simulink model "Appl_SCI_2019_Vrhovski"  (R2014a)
settings: Solver=ode45  StartTime=0.0  StopTime=1000  MaxStep=0.01  RelTol=1e-3
undefined symbols (not defined in the file): deg, H, kg, m, M, mm, N, rad, s, X, Y, Z
libraries: sm_lib x389, nesl_utility x69, simulink x7
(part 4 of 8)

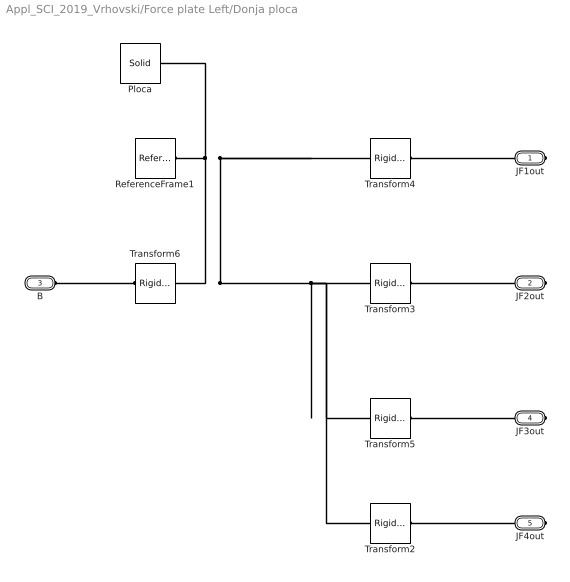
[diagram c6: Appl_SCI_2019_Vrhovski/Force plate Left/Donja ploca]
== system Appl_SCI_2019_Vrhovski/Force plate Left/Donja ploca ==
  Ploca : sm_lib/Body Elements/Solid  InertiaType=Custom  Mass=3.25  MassUnits=kg  CenterOfMass=[0 0 0]  CenterOfMassUnits=mm  MomentsOfInertia=[7450 490 7450]  MomentsOfInertiaUnits=kg*mm^2  ProductsOfInertia=[0 0 0]  ProductsOfInertiaUnits=kg*mm^2  DensityBased=on  Density=1000  DensityUnits=kg/(m^3)  GraphicType=FromGeometry  MarkerShape=Sphere  MarkerSize=10  MarkerSizeUnits=m  GraphicVisPropType=SimpleVisualProperties  GraphicDiffuseColor=[0.6 0.6 0.6]  GraphicSpecularColor=[0.5 0.5 0.5 1.0]  GraphicAmbientColor=[0.15 0.15 0.15 1.0]  GraphicEmissiveColor=[0.0 0.0 0.0 1.0]  GraphicShininess=75  GraphicOpacity=1  GeometryShape=Brick  RectangleSize=[1 1]  RectangleSizeUnits=m  BrickDimensions="[210  380 1]"  BrickDimensionUnits=mm  CylinderRadius=1  CylinderRadiusUnits=m  CylinderLength=1  CylinderLengthUnits=m  SphereRadius=1  SphereRadiusUnits=m  EllipsoidRadii=[1 1 1]  EllipsoidRadiiUnits=m  ExtrusionCrossSection=[1 1; -1 1; -1 -1; 1 -1]  ExtrusionCrossSectionUnits=m  ExtrusionLength=1  ExtrusionLengthUnits=m  PolygonNumSides=3  PolygonOuterRadius=1  PolygonOuterRadiusUnits=m  ExtGeomFileType=STL  ExtGeomFileName=Tijelo_Default_sldprt.STL  ExtGeomFileUnits=mm  RevolutionCrossSection=[1 1; 1 -1; 2 -1; 2 1]  RevolutionCrossSectionUnits=m  RevolutionExtent=Full  RevolutionAngle=180  RevolutionAngleUnits=deg  BlockFunction=simmechanics.library.body_elements.solid
  ReferenceFrame1 : sm_lib/Frames and Transforms/Reference Frame  BlockFunction=simmechanics.library.frames_transforms.reference_frame
  Transform2 : sm_lib/Frames and Transforms/Rigid Transform  TranslationMethod=Cartesian  TranslationLengthUnit=mm  TranslationStandardAxis=+Z  TranslationStandardOffset=15  TranslationCartesianOffset=[84 180.5 1]  TranslationROffset=0  TranslationROffsetUnits=m  TranslationZOffset=0  TranslationZOffsetUnits=m  TranslationThetaOffset=0  TranslationThetaOffsetUnits=deg  RotationMethod=None  RotationAngleUnits=rad  RotationStandardAxis=+Z  RotationAngle=2.0943951023931953  RotationArbitraryAxis=[-0.57735026918962584 -0.57735026918962584 -0.57735026918962584]  FollAlignAxisA=+X  BaseAlignAxisA=+Y  FollAlignAxisB=+Y  BaseAlignAxisB=+Z  BlockFunction=simmechanics.library.frames_transforms.rigid_transform
  Transform3 : sm_lib/Frames and Transforms/Rigid Transform  TranslationMethod=Cartesian  TranslationLengthUnit=mm  TranslationStandardAxis=+Z  TranslationStandardOffset=15  TranslationCartesianOffset=[84 -180.5 1]  TranslationROffset=0  TranslationROffsetUnits=m  TranslationZOffset=0  TranslationZOffsetUnits=m  TranslationThetaOffset=0  TranslationThetaOffsetUnits=deg  RotationMethod=None  RotationAngleUnits=rad  RotationStandardAxis=+Z  RotationAngle=2.0943951023931953  RotationArbitraryAxis=[-0.57735026918962584 -0.57735026918962584 -0.57735026918962584]  FollAlignAxisA=+X  BaseAlignAxisA=+Y  FollAlignAxisB=+Y  BaseAlignAxisB=+Z  BlockFunction=simmechanics.library.frames_transforms.rigid_transform
  Transform4 : sm_lib/Frames and Transforms/Rigid Transform  TranslationMethod=Cartesian  TranslationLengthUnit=mm  TranslationStandardAxis=+Z  TranslationStandardOffset=15  TranslationCartesianOffset=[-84 -180.5 1]  TranslationROffset=0  TranslationROffsetUnits=m  TranslationZOffset=0  TranslationZOffsetUnits=m  TranslationThetaOffset=0  TranslationThetaOffsetUnits=deg  RotationMethod=None  RotationAngleUnits=rad  RotationStandardAxis=+Z  RotationAngle=2.0943951023931953  RotationArbitraryAxis=[-0.57735026918962584 -0.57735026918962584 -0.57735026918962584]  FollAlignAxisA=+X  BaseAlignAxisA=+Y  FollAlignAxisB=+Y  BaseAlignAxisB=+Z  BlockFunction=simmechanics.library.frames_transforms.rigid_transform
  Transform5 : sm_lib/Frames and Transforms/Rigid Transform  TranslationMethod=Cartesian  TranslationLengthUnit=mm  TranslationStandardAxis=+Z  TranslationStandardOffset=15  TranslationCartesianOffset=[-84 180.5 1]  TranslationROffset=0  TranslationROffsetUnits=m  TranslationZOffset=0  TranslationZOffsetUnits=m  TranslationThetaOffset=0  TranslationThetaOffsetUnits=deg  RotationMethod=None  RotationAngleUnits=rad  RotationStandardAxis=+Z  RotationAngle=2.0943951023931953  RotationArbitraryAxis=[-0.57735026918962584 -0.57735026918962584 -0.57735026918962584]  FollAlignAxisA=+X  BaseAlignAxisA=+Y  FollAlignAxisB=+Y  BaseAlignAxisB=+Z  BlockFunction=simmechanics.library.frames_transforms.rigid_transform
  Transform6 : sm_lib/Frames and Transforms/Rigid Transform  TranslationMethod=None  TranslationLengthUnit=mm  TranslationStandardAxis=+Z  TranslationStandardOffset=15  TranslationCartesianOffset="[50  50 15]"  TranslationROffset=0  TranslationROffsetUnits=m  TranslationZOffset=0  TranslationZOffsetUnits=m  TranslationThetaOffset=0  TranslationThetaOffsetUnits=deg  RotationMethod=None  RotationAngleUnits=rad  RotationStandardAxis=+Z  RotationAngle=2.0943951023931953  RotationArbitraryAxis=[-0.57735026918962584 -0.57735026918962584 -0.57735026918962584]  FollAlignAxisA=+X  BaseAlignAxisA=+Y  FollAlignAxisB=+Y  BaseAlignAxisB=+Z  BlockFunction=simmechanics.library.frames_transforms.rigid_transform
  JF1out : PMIOPort  Port=1  Side=Right
  JF2out : PMIOPort  Port=2  Side=Right
  B : PMIOPort  Port=3  Side=Left
  JF3out : PMIOPort  Port=4  Side=Right
  JF4out : PMIOPort  Port=5  Side=Right
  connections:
  JF1out/RConn1 -- Transform4/RConn1
  JF4out/RConn1 -- Transform2/RConn1
  JF3out/RConn1 -- Transform5/RConn1
  ReferenceFrame1/RConn1 -- Ploca/RConn1 -- Transform4/LConn1 -- Transform2/LConn1 -- Transform5/LConn1 -- Transform3/LConn1 -- Transform6/LConn1
  JF2out/RConn1 -- Transform3/RConn1
  B/RConn1 -- Transform6/RConn1

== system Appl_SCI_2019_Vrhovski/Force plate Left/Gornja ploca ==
  Ploca : sm_lib/Body Elements/Solid  InertiaType=Custom  Mass=0  MassUnits=kg  CenterOfMass=[0 0 0]  CenterOfMassUnits=mm  MomentsOfInertia=[7450 490 7450]  MomentsOfInertiaUnits=kg*mm^2  ProductsOfInertia=[0 0 0]  ProductsOfInertiaUnits=kg*mm^2  DensityBased=on  Density=1000  DensityUnits=kg/(m^3)  GraphicType=FromGeometry  MarkerShape=Sphere  MarkerSize=10  MarkerSizeUnits=m  GraphicVisPropType=SimpleVisualProperties  GraphicDiffuseColor=[0.6 0.6 0.6]  GraphicSpecularColor=[0.5 0.5 0.5 1.0]  GraphicAmbientColor=[0.15 0.15 0.15 1.0]  GraphicEmissiveColor=[0.0 0.0 0.0 1.0]  GraphicShininess=75  GraphicOpacity=1  GeometryShape=Brick  RectangleSize=[1 1]  RectangleSizeUnits=m  BrickDimensions="[210  380 1]"  BrickDimensionUnits=mm  CylinderRadius=1  CylinderRadiusUnits=m  CylinderLength=1  CylinderLengthUnits=m  SphereRadius=1  SphereRadiusUnits=m  EllipsoidRadii=[1 1 1]  EllipsoidRadiiUnits=m  ExtrusionCrossSection=[1 1; -1 1; -1 -1; 1 -1]  ExtrusionCrossSectionUnits=m  ExtrusionLength=1  ExtrusionLengthUnits=m  PolygonNumSides=3  PolygonOuterRadius=1  PolygonOuterRadiusUnits=m  ExtGeomFileType=STL  ExtGeomFileName=Tijelo_Default_sldprt.STL  ExtGeomFileUnits=mm  RevolutionCrossSection=[1 1; 1 -1; 2 -1; 2 1]  RevolutionCrossSectionUnits=m  RevolutionExtent=Full  RevolutionAngle=180  RevolutionAngleUnits=deg  BlockFunction=simmechanics.library.body_elements.solid
  ReferenceFrame1 : sm_lib/Frames and Transforms/Reference Frame  BlockFunction=simmechanics.library.frames_transforms.reference_frame
  Transform2 : sm_lib/Frames and Transforms/Rigid Transform  TranslationMethod=None  TranslationLengthUnit=mm  TranslationStandardAxis=+Z  TranslationStandardOffset=15  TranslationCartesianOffset=[50 50 15]  TranslationROffset=0  TranslationROffsetUnits=m  TranslationZOffset=0  TranslationZOffsetUnits=m  TranslationThetaOffset=0  TranslationThetaOffsetUnits=deg  RotationMethod=None  RotationAngleUnits=rad  RotationStandardAxis=+Z  RotationAngle=2.0943951023931953  RotationArbitraryAxis=[-0.57735026918962584 -0.57735026918962584 -0.57735026918962584]  FollAlignAxisA=+X  BaseAlignAxisA=+Y  FollAlignAxisB=+Y  BaseAlignAxisB=+Z  BlockFunction=simmechanics.library.frames_transforms.rigid_transform
  Transform3 : sm_lib/Frames and Transforms/Rigid Transform  TranslationMethod=Cartesian  TranslationLengthUnit=mm  TranslationStandardAxis=+Z  TranslationStandardOffset=15  TranslationCartesianOffset=[84 -180.5 1]  TranslationROffset=0  TranslationROffsetUnits=m  TranslationZOffset=0  TranslationZOffsetUnits=m  TranslationThetaOffset=0  TranslationThetaOffsetUnits=deg  RotationMethod=None  RotationAngleUnits=rad  RotationStandardAxis=+Z  RotationAngle=2.0943951023931953  RotationArbitraryAxis=[-0.57735026918962584 -0.57735026918962584 -0.57735026918962584]  FollAlignAxisA=+X  BaseAlignAxisA=+Y  FollAlignAxisB=+Y  BaseAlignAxisB=+Z  BlockFunction=simmechanics.library.frames_transforms.rigid_transform
  Transform4 : sm_lib/Frames and Transforms/Rigid Transform  TranslationMethod=Cartesian  TranslationLengthUnit=mm  TranslationStandardAxis=+Z  TranslationStandardOffset=15  TranslationCartesianOffset=[-84 -180.5 1]  TranslationROffset=0  TranslationROffsetUnits=m  TranslationZOffset=0  TranslationZOffsetUnits=m  TranslationThetaOffset=0  TranslationThetaOffsetUnits=deg  RotationMethod=None  RotationAngleUnits=rad  RotationStandardAxis=+Z  RotationAngle=2.0943951023931953  RotationArbitraryAxis=[-0.57735026918962584 -0.57735026918962584 -0.57735026918962584]  FollAlignAxisA=+X  BaseAlignAxisA=+Y  FollAlignAxisB=+Y  BaseAlignAxisB=+Z  BlockFunction=simmechanics.library.frames_transforms.rigid_transform
  Transform5 : sm_lib/Frames and Transforms/Rigid Transform  TranslationMethod=Cartesian  TranslationLengthUnit=mm  TranslationStandardAxis=+Z  TranslationStandardOffset=15  TranslationCartesianOffset=[-84 180.5 1]  TranslationROffset=0  TranslationROffsetUnits=m  TranslationZOffset=0  TranslationZOffsetUnits=m  TranslationThetaOffset=0  TranslationThetaOffsetUnits=deg  RotationMethod=None  RotationAngleUnits=rad  RotationStandardAxis=+Z  RotationAngle=2.0943951023931953  RotationArbitraryAxis=[-0.57735026918962584 -0.57735026918962584 -0.57735026918962584]  FollAlignAxisA=+X  BaseAlignAxisA=+Y  FollAlignAxisB=+Y  BaseAlignAxisB=+Z  BlockFunction=simmechanics.library.frames_transforms.rigid_transform
  Transform6 : sm_lib/Frames and Transforms/Rigid Transform  TranslationMethod=Cartesian  TranslationLengthUnit=mm  TranslationStandardAxis=+Z  TranslationStandardOffset=15  TranslationCartesianOffset=[84 180.5 1]  TranslationROffset=0  TranslationROffsetUnits=m  TranslationZOffset=0  TranslationZOffsetUnits=m  TranslationThetaOffset=0  TranslationThetaOffsetUnits=deg  RotationMethod=None  RotationAngleUnits=rad  RotationStandardAxis=+Z  RotationAngle=2.0943951023931953  RotationArbitraryAxis=[-0.57735026918962584 -0.57735026918962584 -0.57735026918962584]  FollAlignAxisA=+X  BaseAlignAxisA=+Y  FollAlignAxisB=+Y  BaseAlignAxisB=+Z  BlockFunction=simmechanics.library.frames_transforms.rigid_transform
  JF1in : PMIOPort  Port=1  Side=Left
  JF2in : PMIOPort  Port=2  Side=Left
  F : PMIOPort  Port=3  Side=Right
  JF3in : PMIOPort  Port=4  Side=Left
  JF4in : PMIOPort  Port=5  Side=Left
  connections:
  F/RConn1 -- Transform2/RConn1
  ReferenceFrame1/RConn1 -- Ploca/RConn1 -- Transform2/LConn1 -- Transform6/LConn1 -- Transform5/LConn1 -- Transform3/LConn1 -- Transform4/LConn1
  JF4in/RConn1 -- Transform6/RConn1
  Transform5/RConn1 -- JF3in/RConn1
  JF2in/RConn1 -- Transform3/RConn1
  Transform4/RConn1 -- JF1in/RConn1

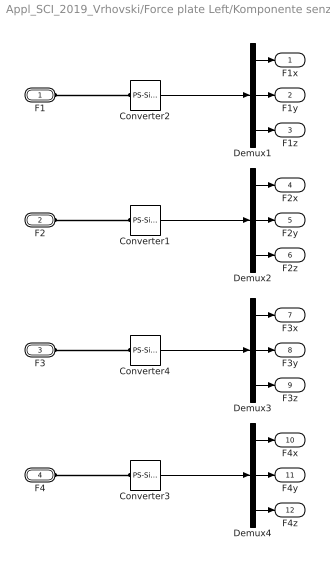
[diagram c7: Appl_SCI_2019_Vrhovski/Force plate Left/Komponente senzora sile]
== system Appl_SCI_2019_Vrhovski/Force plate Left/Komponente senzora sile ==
  Converter{1..4} (4 alike) : nesl_utility/PS-Simulink Converter  PhysicalDomain=network_engine_domain  SubClassName=ps_output  LeftPortType=input  RightPortType=output  PseudoPeriodic=off  Frequencies=[]  Unit=N  AffineConversion=off
  Demux{1..4} (4 alike) : Demux  Outputs=3
  F1 : PMIOPort  Port=1  Side=Left
  F2 : PMIOPort  Port=2  Side=Left
  F3 : PMIOPort  Port=3  Side=Left
  F4 : PMIOPort  Port=4  Side=Left
  F1x : Outport
  F1y : Outport  Port=2
  F1z : Outport  Port=3
  F2x : Outport  Port=4
  F2y : Outport  Port=5
  F2z : Outport  Port=6
  F3x : Outport  Port=7
  F3y : Outport  Port=8
  F3z : Outport  Port=9
  F4x : Outport  Port=10
  F4y : Outport  Port=11
  F4z : Outport  Port=12
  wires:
  Demux1/2 -> F1y/1
  Demux1/1 -> F1x/1
  Demux1/3 -> F1z/1
  Converter2/1 -> Demux1/1
  Demux2/2 -> F2y/1
  Demux2/1 -> F2x/1
  Demux2/3 -> F2z/1
  Converter1/1 -> Demux2/1
  Demux3/2 -> F3y/1
  Demux3/1 -> F3x/1
  Demux3/3 -> F3z/1
  Converter4/1 -> Demux3/1
  Demux4/2 -> F4y/1
  Demux4/1 -> F4x/1
  Demux4/3 -> F4z/1
  Converter3/1 -> Demux4/1
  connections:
  F1/RConn1 -- Converter2/LConn1
  F2/RConn1 -- Converter1/LConn1
  F3/RConn1 -- Converter4/LConn1
  F4/RConn1 -- Converter3/LConn1

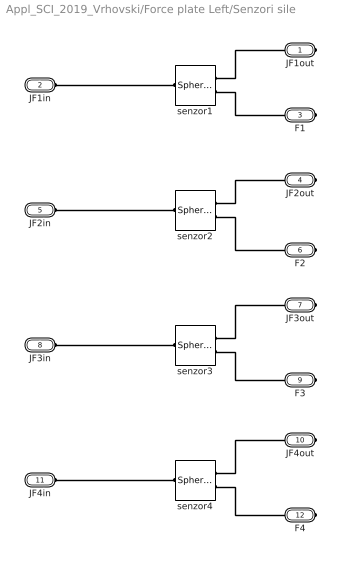
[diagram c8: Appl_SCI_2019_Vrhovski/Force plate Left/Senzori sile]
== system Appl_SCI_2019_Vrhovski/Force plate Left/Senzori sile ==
  senzor{1..4} (4 alike) : sm_lib/Joints/Spherical Joint  SenseConstraintForce=off  SenseConstraintForceX=off  SenseConstraintForceY=off  SenseConstraintForceZ=off  SenseConstraintTorque=off  SenseConstraintTorqueX=off  SenseConstraintTorqueY=off  SenseConstraintTorqueZ=off  SenseTotalForce=on  SenseTotalForceX=off  SenseTotalForceY=off  SenseTotalForceZ=off  SenseTotalTorque=off  SenseTotalTorqueX=off  SenseTotalTorqueY=off  SenseTotalTorqueZ=off  CompositeWrenchDir=FollowerOnBase  CompositeWrenchFrame=BaseFrame  DefPosRotationMethod=None  DefPosRotationAngleUnits=deg  DefPosRotationStandardAxis=+Z  DefPosRotationAngle=0  DefPosRotationArbitraryAxis=[0 0 1]  DefPosFollAlignAxisA=+X  DefPosBaseAlignAxisA=+Y  DefPosFollAlignAxisB=+Y  DefPosBaseAlignAxisB=+Z  EqPosRotationMethod=None  EqPosRotationAngleUnits=deg  EqPosRotationStandardAxis=+Z  EqPosRotationAngle=0  EqPosRotationArbitraryAxis=[0 0 1]  EqPosFollAlignAxisA=+X  EqPosBaseAlignAxisA=+Y  EqPosFollAlignAxisB=+Y  EqPosBaseAlignAxisB=+Z  SpringStiffness=0  SpringStiffnessUnits=m*N/rad  DampingCoefficient=0  DampingCoefficientUnits=m*s*N/rad  ActuateTorqueX=off  ActuateTorqueY=off  ActuateTorqueZ=off  ActuateTorque=off  TorqueActuationMode=NoTorque  MotionActuationMode=ComputedMotion  ActuationFrame=BaseFrame  SensePosition=off  SenseVelocityX=off  SenseVelocityY=off  SenseVelocityZ=off  SenseVelocity=off  SenseAccelerationX=off  SenseAccelerationY=off  SenseAccelerationZ=off  SenseAcceleration=off  SenseTorqueX=off  SenseTorqueY=off  SenseTorqueZ=off  SenseTorqueForce=off  SensingFrame=FollowerFrame  PositionTargetRotationMethod=None  PositionTargetRotationAngleUnits=deg  PositionTargetRotationStandardAxis=+Z  PositionTargetRotationAngle=0  PositionTargetRotationArbitraryAxis=[0 0 1]  PositionTargetFollAlignAxisA=+X  PositionTargetBaseAlignAxisA=+Y  PositionTargetFollAlignAxisB=+Y  PositionTargetBaseAlignAxisB=+Z  PositionTargetSpecify=off  PositionTargetPriority=High  VelocityTargetValue=[0 0 0]  VelocityTargetValueUnits=deg/s  VelocityTargetSpecify=off  VelocityTargetPriority=High  VelocityTargetInFollowerFrame=on  BlockFunction=simmechanics.library.joints.spherical_joint
  JF1out : PMIOPort  Port=1  Side=Right
  JF1in : PMIOPort  Port=2  Side=Left
  F1 : PMIOPort  Port=3  Side=Right
  JF2out : PMIOPort  Port=4  Side=Right
  JF2in : PMIOPort  Port=5  Side=Left
  F2 : PMIOPort  Port=6  Side=Right
  JF3out : PMIOPort  Port=7  Side=Right
  JF3in : PMIOPort  Port=8  Side=Left
  F3 : PMIOPort  Port=9  Side=Right
  JF4out : PMIOPort  Port=10  Side=Right
  JF4in : PMIOPort  Port=11  Side=Left
  F4 : PMIOPort  Port=12  Side=Right
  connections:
  senzor1/RConn1 -- JF1out/RConn1
  senzor3/RConn1 -- JF3out/RConn1
  senzor2/RConn1 -- JF2out/RConn1
  senzor1/RConn2 -- F1/RConn1
  senzor2/RConn2 -- F2/RConn1
  senzor3/RConn2 -- F3/RConn1
  senzor4/RConn2 -- F4/RConn1
  senzor4/RConn1 -- JF4out/RConn1
  senzor1/LConn1 -- JF1in/RConn1
  senzor2/LConn1 -- JF2in/RConn1
  senzor4/LConn1 -- JF4in/RConn1
  senzor3/LConn1 -- JF3in/RConn1

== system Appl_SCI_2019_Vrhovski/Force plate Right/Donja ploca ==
  Ploca : sm_lib/Body Elements/Solid  InertiaType=Custom  Mass=3.25  MassUnits=kg  CenterOfMass=[0 0 0]  CenterOfMassUnits=mm  MomentsOfInertia=[7450 490 7450]  MomentsOfInertiaUnits=kg*mm^2  ProductsOfInertia=[0 0 0]  ProductsOfInertiaUnits=kg*mm^2  DensityBased=on  Density=1000  DensityUnits=kg/(m^3)  GraphicType=FromGeometry  MarkerShape=Sphere  MarkerSize=10  MarkerSizeUnits=m  GraphicVisPropType=SimpleVisualProperties  GraphicDiffuseColor=[0.6 0.6 0.6]  GraphicSpecularColor=[0.5 0.5 0.5 1.0]  GraphicAmbientColor=[0.15 0.15 0.15 1.0]  GraphicEmissiveColor=[0.0 0.0 0.0 1.0]  GraphicShininess=75  GraphicOpacity=1  GeometryShape=Brick  RectangleSize=[1 1]  RectangleSizeUnits=m  BrickDimensions="[210  380 1]"  BrickDimensionUnits=mm  CylinderRadius=1  CylinderRadiusUnits=m  CylinderLength=1  CylinderLengthUnits=m  SphereRadius=1  SphereRadiusUnits=m  EllipsoidRadii=[1 1 1]  EllipsoidRadiiUnits=m  ExtrusionCrossSection=[1 1; -1 1; -1 -1; 1 -1]  ExtrusionCrossSectionUnits=m  ExtrusionLength=1  ExtrusionLengthUnits=m  PolygonNumSides=3  PolygonOuterRadius=1  PolygonOuterRadiusUnits=m  ExtGeomFileType=STL  ExtGeomFileName=Tijelo_Default_sldprt.STL  ExtGeomFileUnits=mm  RevolutionCrossSection=[1 1; 1 -1; 2 -1; 2 1]  RevolutionCrossSectionUnits=m  RevolutionExtent=Full  RevolutionAngle=180  RevolutionAngleUnits=deg  BlockFunction=simmechanics.library.body_elements.solid
  ReferenceFrame1 : sm_lib/Frames and Transforms/Reference Frame  BlockFunction=simmechanics.library.frames_transforms.reference_frame
  Transform2 : sm_lib/Frames and Transforms/Rigid Transform  TranslationMethod=Cartesian  TranslationLengthUnit=mm  TranslationStandardAxis=+Z  TranslationStandardOffset=15  TranslationCartesianOffset=[84 180.5 1]  TranslationROffset=0  TranslationROffsetUnits=m  TranslationZOffset=0  TranslationZOffsetUnits=m  TranslationThetaOffset=0  TranslationThetaOffsetUnits=deg  RotationMethod=None  RotationAngleUnits=rad  RotationStandardAxis=+Z  RotationAngle=2.0943951023931953  RotationArbitraryAxis=[-0.57735026918962584 -0.57735026918962584 -0.57735026918962584]  FollAlignAxisA=+X  BaseAlignAxisA=+Y  FollAlignAxisB=+Y  BaseAlignAxisB=+Z  BlockFunction=simmechanics.library.frames_transforms.rigid_transform
  Transform3 : sm_lib/Frames and Transforms/Rigid Transform  TranslationMethod=Cartesian  TranslationLengthUnit=mm  TranslationStandardAxis=+Z  TranslationStandardOffset=15  TranslationCartesianOffset=[84 -180.5 1]  TranslationROffset=0  TranslationROffsetUnits=m  TranslationZOffset=0  TranslationZOffsetUnits=m  TranslationThetaOffset=0  TranslationThetaOffsetUnits=deg  RotationMethod=None  RotationAngleUnits=rad  RotationStandardAxis=+Z  RotationAngle=2.0943951023931953  RotationArbitraryAxis=[-0.57735026918962584 -0.57735026918962584 -0.57735026918962584]  FollAlignAxisA=+X  BaseAlignAxisA=+Y  FollAlignAxisB=+Y  BaseAlignAxisB=+Z  BlockFunction=simmechanics.library.frames_transforms.rigid_transform
  Transform4 : sm_lib/Frames and Transforms/Rigid Transform  TranslationMethod=Cartesian  TranslationLengthUnit=mm  TranslationStandardAxis=+Z  TranslationStandardOffset=15  TranslationCartesianOffset=[-84 -180.5 1]  TranslationROffset=0  TranslationROffsetUnits=m  TranslationZOffset=0  TranslationZOffsetUnits=m  TranslationThetaOffset=0  TranslationThetaOffsetUnits=deg  RotationMethod=None  RotationAngleUnits=rad  RotationStandardAxis=+Z  RotationAngle=2.0943951023931953  RotationArbitraryAxis=[-0.57735026918962584 -0.57735026918962584 -0.57735026918962584]  FollAlignAxisA=+X  BaseAlignAxisA=+Y  FollAlignAxisB=+Y  BaseAlignAxisB=+Z  BlockFunction=simmechanics.library.frames_transforms.rigid_transform
  Transform5 : sm_lib/Frames and Transforms/Rigid Transform  TranslationMethod=Cartesian  TranslationLengthUnit=mm  TranslationStandardAxis=+Z  TranslationStandardOffset=15  TranslationCartesianOffset=[-84 180.5 1]  TranslationROffset=0  TranslationROffsetUnits=m  TranslationZOffset=0  TranslationZOffsetUnits=m  TranslationThetaOffset=0  TranslationThetaOffsetUnits=deg  RotationMethod=None  RotationAngleUnits=rad  RotationStandardAxis=+Z  RotationAngle=2.0943951023931953  RotationArbitraryAxis=[-0.57735026918962584 -0.57735026918962584 -0.57735026918962584]  FollAlignAxisA=+X  BaseAlignAxisA=+Y  FollAlignAxisB=+Y  BaseAlignAxisB=+Z  BlockFunction=simmechanics.library.frames_transforms.rigid_transform
  Transform6 : sm_lib/Frames and Transforms/Rigid Transform  TranslationMethod=None  TranslationLengthUnit=mm  TranslationStandardAxis=+Z  TranslationStandardOffset=15  TranslationCartesianOffset="[50  50 15]"  TranslationROffset=0  TranslationROffsetUnits=m  TranslationZOffset=0  TranslationZOffsetUnits=m  TranslationThetaOffset=0  TranslationThetaOffsetUnits=deg  RotationMethod=None  RotationAngleUnits=rad  RotationStandardAxis=+Z  RotationAngle=2.0943951023931953  RotationArbitraryAxis=[-0.57735026918962584 -0.57735026918962584 -0.57735026918962584]  FollAlignAxisA=+X  BaseAlignAxisA=+Y  FollAlignAxisB=+Y  BaseAlignAxisB=+Z  BlockFunction=simmechanics.library.frames_transforms.rigid_transform
  JF1out : PMIOPort  Port=1  Side=Right
  JF2out : PMIOPort  Port=2  Side=Right
  B : PMIOPort  Port=3  Side=Left
  JF3out : PMIOPort  Port=4  Side=Right
  JF4out : PMIOPort  Port=5  Side=Right
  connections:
  JF1out/RConn1 -- Transform4/RConn1
  JF4out/RConn1 -- Transform2/RConn1
  JF3out/RConn1 -- Transform5/RConn1
  Transform2/LConn1 -- Transform5/LConn1 -- Transform3/LConn1 -- Transform4/LConn1 -- Ploca/RConn1 -- ReferenceFrame1/RConn1 -- Transform6/LConn1
  JF2out/RConn1 -- Transform3/RConn1
  B/RConn1 -- Transform6/RConn1

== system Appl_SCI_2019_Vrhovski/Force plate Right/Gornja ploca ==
  Ploca : sm_lib/Body Elements/Solid  InertiaType=Custom  Mass=0  MassUnits=kg  CenterOfMass=[0 0 0]  CenterOfMassUnits=mm  MomentsOfInertia=[7450 490 7450]  MomentsOfInertiaUnits=kg*mm^2  ProductsOfInertia=[0 0 0]  ProductsOfInertiaUnits=kg*mm^2  DensityBased=on  Density=1000  DensityUnits=kg/(m^3)  GraphicType=FromGeometry  MarkerShape=Sphere  MarkerSize=10  MarkerSizeUnits=m  GraphicVisPropType=SimpleVisualProperties  GraphicDiffuseColor=[0.6 0.6 0.6]  GraphicSpecularColor=[0.5 0.5 0.5 1.0]  GraphicAmbientColor=[0.15 0.15 0.15 1.0]  GraphicEmissiveColor=[0.0 0.0 0.0 1.0]  GraphicShininess=75  GraphicOpacity=1  GeometryShape=Brick  RectangleSize=[1 1]  RectangleSizeUnits=m  BrickDimensions="[210  380 1]"  BrickDimensionUnits=mm  CylinderRadius=1  CylinderRadiusUnits=m  CylinderLength=1  CylinderLengthUnits=m  SphereRadius=1  SphereRadiusUnits=m  EllipsoidRadii=[1 1 1]  EllipsoidRadiiUnits=m  ExtrusionCrossSection=[1 1; -1 1; -1 -1; 1 -1]  ExtrusionCrossSectionUnits=m  ExtrusionLength=1  ExtrusionLengthUnits=m  PolygonNumSides=3  PolygonOuterRadius=1  PolygonOuterRadiusUnits=m  ExtGeomFileType=STL  ExtGeomFileName=Tijelo_Default_sldprt.STL  ExtGeomFileUnits=mm  RevolutionCrossSection=[1 1; 1 -1; 2 -1; 2 1]  RevolutionCrossSectionUnits=m  RevolutionExtent=Full  RevolutionAngle=180  RevolutionAngleUnits=deg  BlockFunction=simmechanics.library.body_elements.solid
  ReferenceFrame1 : sm_lib/Frames and Transforms/Reference Frame  BlockFunction=simmechanics.library.frames_transforms.reference_frame
  Transform2 : sm_lib/Frames and Transforms/Rigid Transform  TranslationMethod=None  TranslationLengthUnit=mm  TranslationStandardAxis=+Z  TranslationStandardOffset=15  TranslationCartesianOffset=[50 50 15]  TranslationROffset=0  TranslationROffsetUnits=m  TranslationZOffset=0  TranslationZOffsetUnits=m  TranslationThetaOffset=0  TranslationThetaOffsetUnits=deg  RotationMethod=None  RotationAngleUnits=rad  RotationStandardAxis=+Z  RotationAngle=2.0943951023931953  RotationArbitraryAxis=[-0.57735026918962584 -0.57735026918962584 -0.57735026918962584]  FollAlignAxisA=+X  BaseAlignAxisA=+Y  FollAlignAxisB=+Y  BaseAlignAxisB=+Z  BlockFunction=simmechanics.library.frames_transforms.rigid_transform
  Transform3 : sm_lib/Frames and Transforms/Rigid Transform  TranslationMethod=Cartesian  TranslationLengthUnit=mm  TranslationStandardAxis=+Z  TranslationStandardOffset=15  TranslationCartesianOffset=[84 -180.5 1]  TranslationROffset=0  TranslationROffsetUnits=m  TranslationZOffset=0  TranslationZOffsetUnits=m  TranslationThetaOffset=0  TranslationThetaOffsetUnits=deg  RotationMethod=None  RotationAngleUnits=rad  RotationStandardAxis=+Z  RotationAngle=2.0943951023931953  RotationArbitraryAxis=[-0.57735026918962584 -0.57735026918962584 -0.57735026918962584]  FollAlignAxisA=+X  BaseAlignAxisA=+Y  FollAlignAxisB=+Y  BaseAlignAxisB=+Z  BlockFunction=simmechanics.library.frames_transforms.rigid_transform
  Transform4 : sm_lib/Frames and Transforms/Rigid Transform  TranslationMethod=Cartesian  TranslationLengthUnit=mm  TranslationStandardAxis=+Z  TranslationStandardOffset=15  TranslationCartesianOffset=[-84 -180.5 1]  TranslationROffset=0  TranslationROffsetUnits=m  TranslationZOffset=0  TranslationZOffsetUnits=m  TranslationThetaOffset=0  TranslationThetaOffsetUnits=deg  RotationMethod=None  RotationAngleUnits=rad  RotationStandardAxis=+Z  RotationAngle=2.0943951023931953  RotationArbitraryAxis=[-0.57735026918962584 -0.57735026918962584 -0.57735026918962584]  FollAlignAxisA=+X  BaseAlignAxisA=+Y  FollAlignAxisB=+Y  BaseAlignAxisB=+Z  BlockFunction=simmechanics.library.frames_transforms.rigid_transform
  Transform5 : sm_lib/Frames and Transforms/Rigid Transform  TranslationMethod=Cartesian  TranslationLengthUnit=mm  TranslationStandardAxis=+Z  TranslationStandardOffset=15  TranslationCartesianOffset=[-84 180.5 1]  TranslationROffset=0  TranslationROffsetUnits=m  TranslationZOffset=0  TranslationZOffsetUnits=m  TranslationThetaOffset=0  TranslationThetaOffsetUnits=deg  RotationMethod=None  RotationAngleUnits=rad  RotationStandardAxis=+Z  RotationAngle=2.0943951023931953  RotationArbitraryAxis=[-0.57735026918962584 -0.57735026918962584 -0.57735026918962584]  FollAlignAxisA=+X  BaseAlignAxisA=+Y  FollAlignAxisB=+Y  BaseAlignAxisB=+Z  BlockFunction=simmechanics.library.frames_transforms.rigid_transform
  Transform6 : sm_lib/Frames and Transforms/Rigid Transform  TranslationMethod=Cartesian  TranslationLengthUnit=mm  TranslationStandardAxis=+Z  TranslationStandardOffset=15  TranslationCartesianOffset=[84 180.5 1]  TranslationROffset=0  TranslationROffsetUnits=m  TranslationZOffset=0  TranslationZOffsetUnits=m  TranslationThetaOffset=0  TranslationThetaOffsetUnits=deg  RotationMethod=None  RotationAngleUnits=rad  RotationStandardAxis=+Z  RotationAngle=2.0943951023931953  RotationArbitraryAxis=[-0.57735026918962584 -0.57735026918962584 -0.57735026918962584]  FollAlignAxisA=+X  BaseAlignAxisA=+Y  FollAlignAxisB=+Y  BaseAlignAxisB=+Z  BlockFunction=simmechanics.library.frames_transforms.rigid_transform
  JF1in : PMIOPort  Port=1  Side=Left
  JF2in : PMIOPort  Port=2  Side=Left
  F : PMIOPort  Port=3  Side=Right
  JF3in : PMIOPort  Port=4  Side=Left
  JF4in : PMIOPort  Port=5  Side=Left
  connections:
  F/RConn1 -- Transform2/RConn1
  ReferenceFrame1/RConn1 -- Ploca/RConn1 -- Transform2/LConn1 -- Transform6/LConn1 -- Transform5/LConn1 -- Transform3/LConn1 -- Transform4/LConn1
  JF4in/RConn1 -- Transform6/RConn1
  Transform5/RConn1 -- JF3in/RConn1
  JF2in/RConn1 -- Transform3/RConn1
  Transform4/RConn1 -- JF1in/RConn1

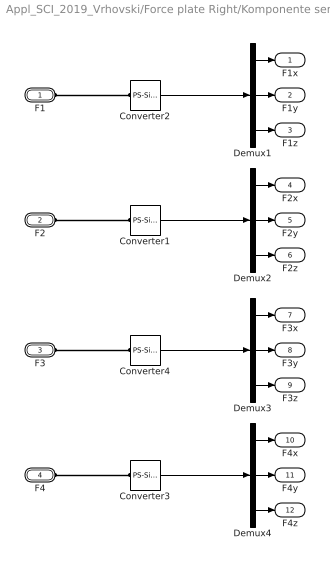
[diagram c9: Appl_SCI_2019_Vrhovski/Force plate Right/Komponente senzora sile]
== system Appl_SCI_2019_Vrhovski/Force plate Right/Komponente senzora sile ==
  Converter{1..4} (4 alike) : nesl_utility/PS-Simulink Converter  PhysicalDomain=network_engine_domain  SubClassName=ps_output  LeftPortType=input  RightPortType=output  PseudoPeriodic=off  Frequencies=[]  Unit=N  AffineConversion=off
  Demux{1..4} (4 alike) : Demux  Outputs=3
  F1 : PMIOPort  Port=1  Side=Left
  F2 : PMIOPort  Port=2  Side=Left
  F3 : PMIOPort  Port=3  Side=Left
  F4 : PMIOPort  Port=4  Side=Left
  F1x : Outport
  F1y : Outport  Port=2
  F1z : Outport  Port=3
  F2x : Outport  Port=4
  F2y : Outport  Port=5
  F2z : Outport  Port=6
  F3x : Outport  Port=7
  F3y : Outport  Port=8
  F3z : Outport  Port=9
  F4x : Outport  Port=10
  F4y : Outport  Port=11
  F4z : Outport  Port=12
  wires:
  Demux1/2 -> F1y/1
  Demux1/1 -> F1x/1
  Demux1/3 -> F1z/1
  Converter2/1 -> Demux1/1
  Demux2/2 -> F2y/1
  Demux2/1 -> F2x/1
  Demux2/3 -> F2z/1
  Converter1/1 -> Demux2/1
  Demux3/2 -> F3y/1
  Demux3/1 -> F3x/1
  Demux3/3 -> F3z/1
  Converter4/1 -> Demux3/1
  Demux4/2 -> F4y/1
  Demux4/1 -> F4x/1
  Demux4/3 -> F4z/1
  Converter3/1 -> Demux4/1
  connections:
  F1/RConn1 -- Converter2/LConn1
  F2/RConn1 -- Converter1/LConn1
  F3/RConn1 -- Converter4/LConn1
  F4/RConn1 -- Converter3/LConn1

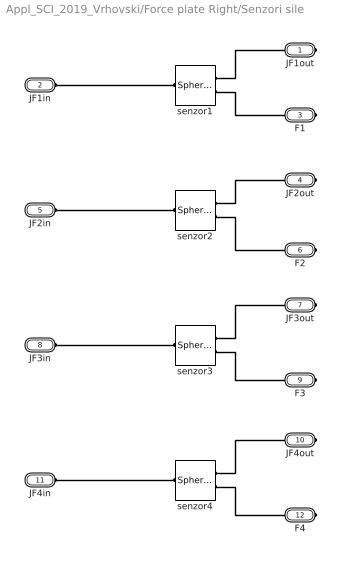
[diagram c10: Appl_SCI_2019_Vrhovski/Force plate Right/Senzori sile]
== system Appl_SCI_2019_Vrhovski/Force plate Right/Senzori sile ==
  senzor{1..4} (4 alike) : sm_lib/Joints/Spherical Joint  SenseConstraintForce=off  SenseConstraintForceX=off  SenseConstraintForceY=off  SenseConstraintForceZ=off  SenseConstraintTorque=off  SenseConstraintTorqueX=off  SenseConstraintTorqueY=off  SenseConstraintTorqueZ=off  SenseTotalForce=on  SenseTotalForceX=off  SenseTotalForceY=off  SenseTotalForceZ=off  SenseTotalTorque=off  SenseTotalTorqueX=off  SenseTotalTorqueY=off  SenseTotalTorqueZ=off  CompositeWrenchDir=FollowerOnBase  CompositeWrenchFrame=BaseFrame  DefPosRotationMethod=None  DefPosRotationAngleUnits=deg  DefPosRotationStandardAxis=+Z  DefPosRotationAngle=0  DefPosRotationArbitraryAxis=[0 0 1]  DefPosFollAlignAxisA=+X  DefPosBaseAlignAxisA=+Y  DefPosFollAlignAxisB=+Y  DefPosBaseAlignAxisB=+Z  EqPosRotationMethod=None  EqPosRotationAngleUnits=deg  EqPosRotationStandardAxis=+Z  EqPosRotationAngle=0  EqPosRotationArbitraryAxis=[0 0 1]  EqPosFollAlignAxisA=+X  EqPosBaseAlignAxisA=+Y  EqPosFollAlignAxisB=+Y  EqPosBaseAlignAxisB=+Z  SpringStiffness=0  SpringStiffnessUnits=m*N/rad  DampingCoefficient=0  DampingCoefficientUnits=m*s*N/rad  ActuateTorqueX=off  ActuateTorqueY=off  ActuateTorqueZ=off  ActuateTorque=off  TorqueActuationMode=NoTorque  MotionActuationMode=ComputedMotion  ActuationFrame=BaseFrame  SensePosition=off  SenseVelocityX=off  SenseVelocityY=off  SenseVelocityZ=off  SenseVelocity=off  SenseAccelerationX=off  SenseAccelerationY=off  SenseAccelerationZ=off  SenseAcceleration=off  SenseTorqueX=off  SenseTorqueY=off  SenseTorqueZ=off  SenseTorqueForce=off  SensingFrame=FollowerFrame  PositionTargetRotationMethod=None  PositionTargetRotationAngleUnits=deg  PositionTargetRotationStandardAxis=+Z  PositionTargetRotationAngle=0  PositionTargetRotationArbitraryAxis=[0 0 1]  PositionTargetFollAlignAxisA=+X  PositionTargetBaseAlignAxisA=+Y  PositionTargetFollAlignAxisB=+Y  PositionTargetBaseAlignAxisB=+Z  PositionTargetSpecify=off  PositionTargetPriority=High  VelocityTargetValue=[0 0 0]  VelocityTargetValueUnits=deg/s  VelocityTargetSpecify=off  VelocityTargetPriority=High  VelocityTargetInFollowerFrame=on  BlockFunction=simmechanics.library.joints.spherical_joint
  JF1out : PMIOPort  Port=1  Side=Right
  JF1in : PMIOPort  Port=2  Side=Left
  F1 : PMIOPort  Port=3  Side=Right
  JF2out : PMIOPort  Port=4  Side=Right
  JF2in : PMIOPort  Port=5  Side=Left
  F2 : PMIOPort  Port=6  Side=Right
  JF3out : PMIOPort  Port=7  Side=Right
  JF3in : PMIOPort  Port=8  Side=Left
  F3 : PMIOPort  Port=9  Side=Right
  JF4out : PMIOPort  Port=10  Side=Right
  JF4in : PMIOPort  Port=11  Side=Left
  F4 : PMIOPort  Port=12  Side=Right
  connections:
  senzor1/RConn1 -- JF1out/RConn1
  senzor3/RConn1 -- JF3out/RConn1
  senzor2/RConn1 -- JF2out/RConn1
  senzor1/RConn2 -- F1/RConn1
  senzor2/RConn2 -- F2/RConn1
  senzor3/RConn2 -- F3/RConn1
  senzor4/RConn2 -- F4/RConn1
  senzor4/RConn1 -- JF4out/RConn1
  senzor1/LConn1 -- JF1in/RConn1
  senzor2/LConn1 -- JF2in/RConn1
  senzor4/LConn1 -- JF4in/RConn1
  senzor3/LConn1 -- JF3in/RConn1

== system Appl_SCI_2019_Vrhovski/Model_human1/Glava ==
  ReferenceFrame : sm_lib/Frames and Transforms/Reference Frame  BlockFunction=simmechanics.library.frames_transforms.reference_frame
  Solid : sm_lib/Body Elements/Solid  InertiaType=Custom  Mass=0.05625*M  MassUnits=kg  CenterOfMass=[0 0 0]  CenterOfMassUnits=mm  MomentsOfInertia=[2897.1863857204326 1.8962829928219973 2897.1862300567827]  MomentsOfInertiaUnits=kg*mm^2  ProductsOfInertia=[0 0 -0.00027890183916846033]  ProductsOfInertiaUnits=kg*mm^2  DensityBased=on  Density=1000  DensityUnits=kg/(m^3)  GraphicType=FromGeometry  MarkerShape=Sphere  MarkerSize=10  MarkerSizeUnits=m  GraphicVisPropType=SimpleVisualProperties  GraphicDiffuseColor=[0.792156862745098 0.81960784313725488 0.93333333333333335]  GraphicSpecularColor=[0.5 0.5 0.5 1.0]  GraphicAmbientColor=[0.15 0.15 0.15 1.0]  GraphicEmissiveColor=[0.0 0.0 0.0 1.0]  GraphicShininess=75  GraphicOpacity=1  GeometryShape=Sphere  RectangleSize=[1 1]  RectangleSizeUnits=m  BrickDimensions=[1 1 1]  BrickDimensionUnits=m  CylinderRadius=1  CylinderRadiusUnits=m  CylinderLength=1  CylinderLengthUnits=m  SphereRadius=9  SphereRadiusUnits=cm  EllipsoidRadii=[1 1 1]  EllipsoidRadiiUnits=m  ExtrusionCrossSection=[1 1; -1 1; -1 -1; 1 -1]  ExtrusionCrossSectionUnits=m  ExtrusionLength=1  ExtrusionLengthUnits=m  PolygonNumSides=3  PolygonOuterRadius=1  PolygonOuterRadiusUnits=m  ExtGeomFileType=STL  ExtGeomFileName=Pod_Default_sldprt.STL  ExtGeomFileUnits=mm  RevolutionCrossSection=[1 1; 1 -1; 2 -1; 2 1]  RevolutionCrossSectionUnits=m  RevolutionExtent=Full  RevolutionAngle=180  RevolutionAngleUnits=deg  BlockFunction=simmechanics.library.body_elements.solid
  Transform : sm_lib/Frames and Transforms/Rigid Transform  TranslationMethod=None  TranslationLengthUnit=mm  TranslationStandardAxis=+Z  TranslationStandardOffset=0  TranslationCartesianOffset=[-2.2026824808563106e-13 549.99999999999943 3.4106051316484809e-13]  TranslationROffset=0  TranslationROffsetUnits=m  TranslationZOffset=0  TranslationZOffsetUnits=m  TranslationThetaOffset=0  TranslationThetaOffsetUnits=deg  RotationMethod=None  RotationAngleUnits=rad  RotationStandardAxis=+Z  RotationAngle=2.0943951023931962  RotationArbitraryAxis=[0.57735026918962595 -0.57735026918962618 0.57735026918962518]  FollAlignAxisA=+X  BaseAlignAxisA=+Y  FollAlignAxisB=+Y  BaseAlignAxisB=+Z  BlockFunction=simmechanics.library.frames_transforms.rigid_transform
  Transform1 : sm_lib/Frames and Transforms/Rigid Transform  TranslationMethod=None  TranslationLengthUnit=mm  TranslationStandardAxis=+Z  TranslationStandardOffset=0  TranslationCartesianOffset=[1.3358203432289883e-12 650.00000000000045 -1.0913936421275139e-11]  TranslationROffset=0  TranslationROffsetUnits=m  TranslationZOffset=0  TranslationZOffsetUnits=m  TranslationThetaOffset=0  TranslationThetaOffsetUnits=deg  RotationMethod=None  RotationAngleUnits=rad  RotationStandardAxis=+Z  RotationAngle=0  RotationArbitraryAxis=[0 0 0]  FollAlignAxisA=+X  BaseAlignAxisA=+Y  FollAlignAxisB=+Y  BaseAlignAxisB=+Z  BlockFunction=simmechanics.library.frames_transforms.rigid_transform
  F : PMIOPort  Port=1  Side=Right
  B : PMIOPort  Port=2  Side=Left
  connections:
  Transform/LConn1 -- Transform1/LConn1 -- ReferenceFrame/RConn1 -- Solid/RConn1
  Transform/RConn1 -- B/RConn1
  Transform1/RConn1 -- F/RConn1

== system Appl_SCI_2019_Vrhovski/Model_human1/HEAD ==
  Mux : Mux  Inputs=3
  Pos X Converter : nesl_utility/PS-Simulink Converter  PhysicalDomain=network_engine_domain  SubClassName=ps_output  LeftPortType=input  RightPortType=output  PseudoPeriodic=off  Frequencies=[]  Unit=mm  AffineConversion=off
  Pos Y Converter : nesl_utility/PS-Simulink Converter  PhysicalDomain=network_engine_domain  SubClassName=ps_output  LeftPortType=input  RightPortType=output  PseudoPeriodic=off  Frequencies=[]  Unit=mm  AffineConversion=off
  Pos Z Converter2 : nesl_utility/PS-Simulink Converter  PhysicalDomain=network_engine_domain  SubClassName=ps_output  LeftPortType=input  RightPortType=output  PseudoPeriodic=off  Frequencies=[]  Unit=mm  AffineConversion=off
  Transform Sensor : sm_lib/Frames and Transforms/Transform Sensor  MeasurementFrame=World  SenseAngle=off  SenseAxis=off  SenseAngle1=off  SenseAngle2=off  SenseAngle3=off  SenseQ=off  SenseR=off  SenseOmegaX=off  SenseOmegaY=off  SenseOmegaZ=off  SenseOmega1=off  SenseOmega2=off  SenseOmega3=off  SenseQDot=off  SenseRDot=off  SenseAlphaX=off  SenseAlphaY=off  SenseAlphaZ=off  SenseAlpha1=off  SenseAlpha2=off  SenseAlpha3=off  SenseQDDot=off  SenseRDDot=off  SenseX=on  SenseY=on  SenseZ=on  SenseRad=on  SenseAzim=off  SenseDist=off  SenseInc=off  SenseXDot=off  SenseYDot=off  SenseZDot=off  SenseRadDot=off  SenseAzimDot=off  SenseDistDot=off  SenseIncDot=off  SenseXDDot=off  SenseYDDot=off  SenseZDDot=off  SenseRadDDot=off  SenseAzimDDot=off  SenseDistDDot=off  SenseIncDDot=off  BlockFunction=simmechanics.library.frames_transforms.transform_sensor
  base_coord_sys : PMIOPort  Port=1  Side=Left
  marker : PMIOPort  Port=2  Side=Left
  xyz : Outport
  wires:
  Mux/1 -> xyz/1
  Pos Y Converter/1 -> Mux/2
  Pos X Converter/1 -> Mux/1
  Pos Z Converter2/1 -> Mux/3
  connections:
  Transform Sensor/RConn3 -- Pos Y Converter/LConn1
  Pos X Converter/LConn1 -- Transform Sensor/RConn2
  Pos Z Converter2/LConn1 -- Transform Sensor/RConn4
  marker/RConn1 -- Transform Sensor/RConn1
  base_coord_sys/RConn1 -- Transform Sensor/LConn1

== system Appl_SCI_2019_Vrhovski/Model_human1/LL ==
  L1 : Subsystem
  L2 : Subsystem
  L3 : Subsystem
  B : PMIOPort  Port=1  Side=Left
  FL1 : PMIOPort  Port=2  Side=Left
  FL2 : PMIOPort  Port=3  Side=Left
  FL3 : PMIOPort  Port=4  Side=Left
  Lxyz1 : Outport
  Lxyz2 : Outport  Port=2
  Lxyz3 : Outport  Port=3
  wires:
  L1/1(xyz) -> Lxyz1/1
  L3/1(xyz) -> Lxyz3/1
  L2/1(xyz) -> Lxyz2/1
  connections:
  L1/LConn1 -- B/RConn1 -- L2/LConn1 -- L3/LConn1
  L3/LConn2 -- FL3/RConn1
  L1/LConn2 -- FL1/RConn1
  FL2/RConn1 -- L2/LConn2

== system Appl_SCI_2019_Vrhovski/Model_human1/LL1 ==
  L1 : Subsystem
  L2 : Subsystem
  L3 : Subsystem
  B : PMIOPort  Port=1  Side=Left
  FL1 : PMIOPort  Port=2  Side=Left
  FL2 : PMIOPort  Port=3  Side=Left
  FL3 : PMIOPort  Port=4  Side=Left
  Lxyz1 : Outport
  Lxyz2 : Outport  Port=2
  Lxyz3 : Outport  Port=3
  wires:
  L2/1(xyz) -> Lxyz2/1
  L3/1(xyz) -> Lxyz3/1
  L1/1(xyz) -> Lxyz1/1
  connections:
  FL2/RConn1 -- L2/LConn2
  L1/LConn2 -- FL1/RConn1
  L3/LConn2 -- FL3/RConn1
  B/RConn1 -- L1/LConn1 -- L3/LConn1 -- L2/LConn1

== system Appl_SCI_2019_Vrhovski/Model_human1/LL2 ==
  L1 : Subsystem
  L2 : Subsystem
  L3 : Subsystem
  B : PMIOPort  Port=1  Side=Left
  FL1 : PMIOPort  Port=2  Side=Left
  FL2 : PMIOPort  Port=3  Side=Left
  FL3 : PMIOPort  Port=4  Side=Left
  Lxyz1 : Outport
  Lxyz2 : Outport  Port=2
  Lxyz3 : Outport  Port=3
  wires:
  L1/1(xyz) -> Lxyz1/1
  L3/1(xyz) -> Lxyz3/1
  L2/1(xyz) -> Lxyz2/1
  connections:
  L2/LConn1 -- L3/LConn1 -- L1/LConn1 -- B/RConn1
  L3/LConn2 -- FL3/RConn1
  L1/LConn2 -- FL1/RConn1
  FL2/RConn1 -- L2/LConn2

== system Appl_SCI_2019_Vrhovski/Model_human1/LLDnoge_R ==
  Cylindrical1 : sm_lib/Joints/Cylindrical Joint  SenseConstraintForce=off  SenseConstraintForceX=off  SenseConstraintForceY=off  SenseConstraintForceZ=off  SenseConstraintTorque=off  SenseConstraintTorqueX=off  SenseConstraintTorqueY=off  SenseConstraintTorqueZ=off  SenseTotalForce=off  SenseTotalForceX=off  SenseTotalForceY=off  SenseTotalForceZ=off  SenseTotalTorque=off  SenseTotalTorqueX=off  SenseTotalTorqueY=off  SenseTotalTorqueZ=off  CompositeWrenchDir=FollowerOnBase  CompositeWrenchFrame=BaseFrame  PzEquilibriumPosition=0  PzEquilibriumPositionUnits=m  PzSpringStiffness=0  PzSpringStiffnessUnits=N/m  PzDampingCoefficient=0  PzDampingCoefficientUnits=s*N/m  PzTorqueActuationMode=ComputedTorque  PzMotionActuationMode=InputMotion  PzSensePosition=off  PzSenseVelocity=off  PzSenseAcceleration=off  PzSenseTorqueForce=off  PzPositionTargetValue=0  PzPositionTargetValueUnits=mm  PzPositionTargetSpecify=on  PzPositionTargetPriority=Low  PzVelocityTargetValue=0  PzVelocityTargetValueUnits=m/s  PzVelocityTargetSpecify=off  PzVelocityTargetPriority=High  RzEquilibriumPosition=0  RzEquilibriumPositionUnits=rad  RzSpringStiffness=0  RzSpringStiffnessUnits=m*N/rad  RzDampingCoefficient=0  RzDampingCoefficientUnits=m*s*N/rad  RzTorqueActuationMode=NoTorque  RzMotionActuationMode=ComputedMotion  RzSensePosition=off  RzSenseVelocity=off  RzSenseAcceleration=off  RzSenseTorqueForce=off  RzPositionTargetValue=28.897330136086104  RzPositionTargetValueUnits=deg  RzPositionTargetSpecify=off  RzPositionTargetPriority=Low  RzVelocityTargetValue=0  RzVelocityTargetValueUnits=deg/s  RzVelocityTargetSpecify=off  RzVelocityTargetPriority=High  BlockFunction=simmechanics.library.joints.cylindrical_joint
  LLD_R : Subsystem
  Transform1 : sm_lib/Frames and Transforms/Rigid Transform  TranslationMethod=StandardAxis  TranslationLengthUnit=mm  TranslationStandardAxis=-Z  TranslationStandardOffset=100  TranslationCartesianOffset=[1.3358203432289883e-12 650.00000000000045 -1.0913936421275139e-11]  TranslationROffset=0  TranslationROffsetUnits=m  TranslationZOffset=0  TranslationZOffsetUnits=m  TranslationThetaOffset=0  TranslationThetaOffsetUnits=deg  RotationMethod=None  RotationAngleUnits=rad  RotationStandardAxis=+Z  RotationAngle=0  RotationArbitraryAxis=[0 0 0]  FollAlignAxisA=+X  BaseAlignAxisA=+Y  FollAlignAxisB=+Y  BaseAlignAxisB=+Z  BlockFunction=simmechanics.library.frames_transforms.rigid_transform
  Transform2 : sm_lib/Frames and Transforms/Rigid Transform  TranslationMethod=StandardAxis  TranslationLengthUnit=mm  TranslationStandardAxis=+Z  TranslationStandardOffset=100  TranslationCartesianOffset=[1.3358203432289883e-12 650.00000000000045 -1.0913936421275139e-11]  TranslationROffset=0  TranslationROffsetUnits=m  TranslationZOffset=0  TranslationZOffsetUnits=m  TranslationThetaOffset=0  TranslationThetaOffsetUnits=deg  RotationMethod=None  RotationAngleUnits=rad  RotationStandardAxis=+Z  RotationAngle=0  RotationArbitraryAxis=[0 0 0]  FollAlignAxisA=+X  BaseAlignAxisA=+Y  FollAlignAxisB=+Y  BaseAlignAxisB=+Z  BlockFunction=simmechanics.library.frames_transforms.rigid_transform
  B : PMIOPort  Port=1  Side=Left
  F : PMIOPort  Port=2  Side=Right
  LLD : PMIOPort  Port=3  Side=Left
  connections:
  LLD/RConn1 -- Cylindrical1/LConn2
  B/RConn1 -- Transform1/LConn1
  Transform1/RConn1 -- Cylindrical1/LConn1
  LLD_R/LConn1 -- Cylindrical1/RConn1
  Transform2/RConn1 -- F/RConn1
  Transform2/LConn1 -- LLD_R/RConn1

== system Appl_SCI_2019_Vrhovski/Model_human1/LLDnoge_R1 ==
  Cylindrical1 : sm_lib/Joints/Cylindrical Joint  SenseConstraintForce=off  SenseConstraintForceX=off  SenseConstraintForceY=off  SenseConstraintForceZ=off  SenseConstraintTorque=off  SenseConstraintTorqueX=off  SenseConstraintTorqueY=off  SenseConstraintTorqueZ=off  SenseTotalForce=off  SenseTotalForceX=off  SenseTotalForceY=off  SenseTotalForceZ=off  SenseTotalTorque=off  SenseTotalTorqueX=off  SenseTotalTorqueY=off  SenseTotalTorqueZ=off  CompositeWrenchDir=FollowerOnBase  CompositeWrenchFrame=BaseFrame  PzEquilibriumPosition=0  PzEquilibriumPositionUnits=m  PzSpringStiffness=0  PzSpringStiffnessUnits=N/m  PzDampingCoefficient=0  PzDampingCoefficientUnits=s*N/m  PzTorqueActuationMode=ComputedTorque  PzMotionActuationMode=InputMotion  PzSensePosition=off  PzSenseVelocity=off  PzSenseAcceleration=off  PzSenseTorqueForce=off  PzPositionTargetValue=0  PzPositionTargetValueUnits=mm  PzPositionTargetSpecify=on  PzPositionTargetPriority=Low  PzVelocityTargetValue=0  PzVelocityTargetValueUnits=m/s  PzVelocityTargetSpecify=off  PzVelocityTargetPriority=High  RzEquilibriumPosition=0  RzEquilibriumPositionUnits=rad  RzSpringStiffness=0  RzSpringStiffnessUnits=m*N/rad  RzDampingCoefficient=0  RzDampingCoefficientUnits=m*s*N/rad  RzTorqueActuationMode=NoTorque  RzMotionActuationMode=ComputedMotion  RzSensePosition=off  RzSenseVelocity=off  RzSenseAcceleration=off  RzSenseTorqueForce=off  RzPositionTargetValue=28.897330136086104  RzPositionTargetValueUnits=deg  RzPositionTargetSpecify=off  RzPositionTargetPriority=Low  RzVelocityTargetValue=0  RzVelocityTargetValueUnits=deg/s  RzVelocityTargetSpecify=off  RzVelocityTargetPriority=High  BlockFunction=simmechanics.library.joints.cylindrical_joint
  LLD_R : Subsystem
  Transform1 : sm_lib/Frames and Transforms/Rigid Transform  TranslationMethod=StandardAxis  TranslationLengthUnit=mm  TranslationStandardAxis=-Z  TranslationStandardOffset=100  TranslationCartesianOffset=[1.3358203432289883e-12 650.00000000000045 -1.0913936421275139e-11]  TranslationROffset=0  TranslationROffsetUnits=m  TranslationZOffset=0  TranslationZOffsetUnits=m  TranslationThetaOffset=0  TranslationThetaOffsetUnits=deg  RotationMethod=None  RotationAngleUnits=rad  RotationStandardAxis=+Z  RotationAngle=0  RotationArbitraryAxis=[0 0 0]  FollAlignAxisA=+X  BaseAlignAxisA=+Y  FollAlignAxisB=+Y  BaseAlignAxisB=+Z  BlockFunction=simmechanics.library.frames_transforms.rigid_transform
  Transform2 : sm_lib/Frames and Transforms/Rigid Transform  TranslationMethod=StandardAxis  TranslationLengthUnit=mm  TranslationStandardAxis=+Z  TranslationStandardOffset=100  TranslationCartesianOffset=[1.3358203432289883e-12 650.00000000000045 -1.0913936421275139e-11]  TranslationROffset=0  TranslationROffsetUnits=m  TranslationZOffset=0  TranslationZOffsetUnits=m  TranslationThetaOffset=0  TranslationThetaOffsetUnits=deg  RotationMethod=None  RotationAngleUnits=rad  RotationStandardAxis=+Z  RotationAngle=0  RotationArbitraryAxis=[0 0 0]  FollAlignAxisA=+X  BaseAlignAxisA=+Y  FollAlignAxisB=+Y  BaseAlignAxisB=+Z  BlockFunction=simmechanics.library.frames_transforms.rigid_transform
  B : PMIOPort  Port=1  Side=Left
  F : PMIOPort  Port=2  Side=Right
  LLD : PMIOPort  Port=3  Side=Left
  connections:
  Transform2/LConn1 -- LLD_R/RConn1
  Transform2/RConn1 -- F/RConn1
  LLD_R/LConn1 -- Cylindrical1/RConn1
  Transform1/RConn1 -- Cylindrical1/LConn1
  B/RConn1 -- Transform1/LConn1
  LLD/RConn1 -- Cylindrical1/LConn2

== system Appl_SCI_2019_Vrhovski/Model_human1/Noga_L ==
  koljeno : Subsystem
  natkoljenica : Subsystem
  potkoljenica : Subsystem
  skocni_zglob_L : Subsystem
  skocni_zglob_L Joint : sm_lib/Joints/Universal Joint  SenseConstraintForce=off  SenseConstraintForceX=off  SenseConstraintForceY=off  SenseConstraintForceZ=off  SenseConstraintTorque=off  SenseConstraintTorqueX=off  SenseConstraintTorqueY=off  SenseConstraintTorqueZ=off  SenseTotalForce=off  SenseTotalForceX=off  SenseTotalForceY=off  SenseTotalForceZ=off  SenseTotalTorque=off  SenseTotalTorqueX=off  SenseTotalTorqueY=off  SenseTotalTorqueZ=off  CompositeWrenchDir=FollowerOnBase  CompositeWrenchFrame=BaseFrame  RxEquilibriumPosition=0  RxEquilibriumPositionUnits=deg  RxSpringStiffness=0  RxSpringStiffnessUnits=N*m/deg  RxDampingCoefficient=0  RxDampingCoefficientUnits=N*m/(deg/s)  RxTorqueActuationMode=NoTorque  RxMotionActuationMode=ComputedMotion  RxSensePosition=off  RxSenseVelocity=off  RxSenseAcceleration=off  RxSenseTorqueForce=off  RxPositionTargetValue=0  RxPositionTargetValueUnits=deg  RxPositionTargetSpecify=off  RxPositionTargetPriority=High  RxVelocityTargetValue=0  RxVelocityTargetValueUnits=deg/s  RxVelocityTargetSpecify=off  RxVelocityTargetPriority=High  RyEquilibriumPosition=0  RyEquilibriumPositionUnits=deg  RySpringStiffness=0  RySpringStiffnessUnits=N*m/deg  RyDampingCoefficient=0  RyDampingCoefficientUnits=N*m/(deg/s)  RyTorqueActuationMode=NoTorque  RyMotionActuationMode=ComputedMotion  RySensePosition=off  RySenseVelocity=off  RySenseAcceleration=off  RySenseTorqueForce=off  RyPositionTargetValue=0  RyPositionTargetValueUnits=deg  RyPositionTargetSpecify=off  RyPositionTargetPriority=High  RyVelocityTargetValue=0  RyVelocityTargetValueUnits=deg/s  RyVelocityTargetSpecify=off  RyVelocityTargetPriority=High  BlockFunction=simmechanics.library.joints.universal_joint
  B : PMIOPort  Port=1  Side=Left
  F : PMIOPort  Port=2  Side=Right
  LL1 : PMIOPort  Port=3  Side=Right
  LL2 : PMIOPort  Port=4  Side=Right
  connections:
  B/RConn1 -- skocni_zglob_L/LConn1
  skocni_zglob_L/RConn1 -- LL1/RConn1 -- skocni_zglob_L Joint/LConn1
  potkoljenica/LConn1 -- skocni_zglob_L Joint/RConn1
  natkoljenica/LConn1 -- LL2/RConn1 -- koljeno/RConn1
  koljeno/LConn1 -- potkoljenica/RConn1
  F/RConn1 -- natkoljenica/RConn1
